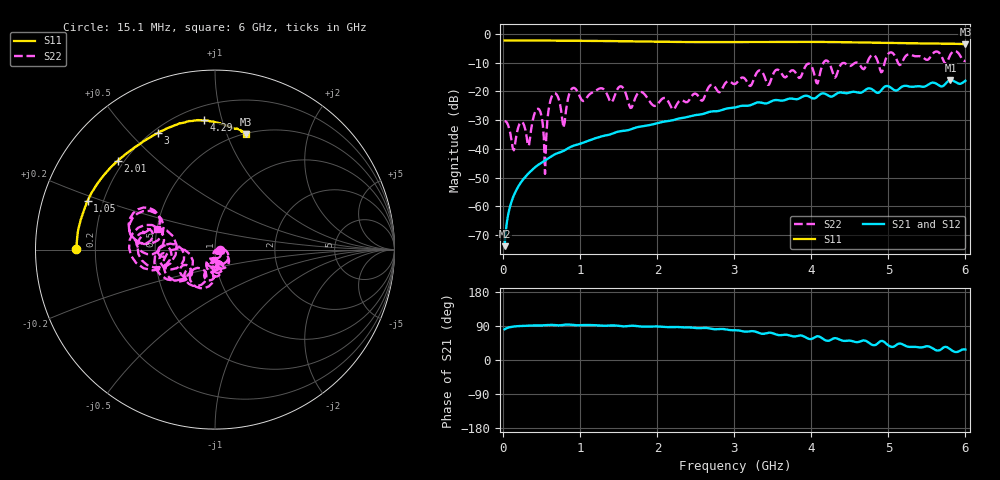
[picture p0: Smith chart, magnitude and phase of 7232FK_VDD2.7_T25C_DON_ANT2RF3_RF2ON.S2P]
!Agilent Technologies,E5071C,MY46417908,A.11.23
!Date: Fri Mar 03 11:28:58 2017
!Data & Calibration Information:
!Freq	S11:SOLT2(ON)	S21:SOLT2(ON)	S12:SOLT2(ON)	S22:SOLT2(ON)
!PortZ  Port1:50+j0  Port2:50+j0
!Above PortZ is port z conversion or system Z0 setting when saving the data.
!When reading, reference impedance value at option line is always used.
# Hz S dB R 50
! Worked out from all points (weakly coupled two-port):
!   400 points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, 15.1 MHz to 6 GHz, reference 50 ohm
!   highest |S21| = -16.12 dB at 5.805 GHz (marker M1); lowest = -73.8 dB at 15.1 MHz (marker M2)
!   lowest |S11| = -3.5 dB at 6 GHz (marker M3), VSWR 4.98, Z = 25.5 + j58.7 ohm
!   |S11| at or under -10 dB: nowhere
!   |S22| runs from -48.7 to -5.9 dB; largest |S21 - S12| = 0.0028
!   S11 on the Smith chart (normalised r, x): 15.1 MHz: 0.13, +0.00; 1.05 GHz: 0.14, +0.18; 2.01 GHz: 0.18, +0.38; 3 GHz: 0.22, +0.60; 4.29 GHz: 0.29, +0.88; 6 GHz: 0.51, +1.17
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1.509975e7  -2.25 179.7  -73.84 81.1  -73.81 80.5  -30.28 -9.3
1.050982e8  -2.26 178.1  -58.33 87.5  -58.34 87.4  -37.03 -60.1
2.40096e8  -2.26 175.5  -51.16 89.7  -51.16 89.8  -30.63 -48.4
3.300945e8  -2.27 173.9  -48.40 90.8  -48.39 90.8  -38.92 -34.9
4.650922e8  -2.28 171.5  -45.30 91.1  -45.29 91.1  -26.29 -80.8
5.100915e8  -2.28 170.7  -44.53 91.5  -44.52 91.5  -31.22 -110.4
5.40091e8  -2.29 170.1  -44.02 91.8  -44.03 91.8  -48.69 -62.8
5.700905e8  -2.29 169.5  -43.51 92.5  -43.51 92.6  -30.09 12.5
6.300895e8  -2.31 168.3  -42.47 92.7  -42.47 92.7  -21.58 -25.2
7.80087e8  -2.34 165.1  -40.69 92.8  -40.70 92.8  -32.65 -64.4
8.850852e8  -2.36 162.7  -39.15 92.9  -39.16 92.9  -19.14 -47.5
1.020083e9  -2.37 159.7  -37.97 92.1  -37.99 92.1  -23.09 -79.0
1.050082e9  -2.38 159.1  -37.67 92.4  -37.69 92.3  -23.16 -70.6
2.010066e9  -2.69 137.7  -30.95 88.4  -30.96 88.4  -24.18 -94.1
3.00005e9  -2.80 116.0  -25.62 78.6  -25.62 78.7  -17.44 -93.9
3.01505e9  -2.80 115.7  -25.53 78.6  -25.52 78.6  -17.33 -92.3
4.005033e9  -2.76 98.6  -22.29 55.8  -22.27 55.6  -11.39 -174.6
4.290028e9  -2.82 94.8  -21.48 57.1  -21.51 56.9  -14.58 178.4
4.905018e9  -3.08 87.5  -19.66 50.2  -19.68 50.0  -13.33 173.2
5.010016e9  -3.10 86.8  -18.31 37.2  -18.23 37.4  -6.59 -175.7
5.805003e9  -3.41 77.5  -16.12 28.0  -16.11 28.8  -7.20 173.9
6e9  -3.54 74.8  -16.29 27.6  -16.32 28.4  -9.26 160.9
